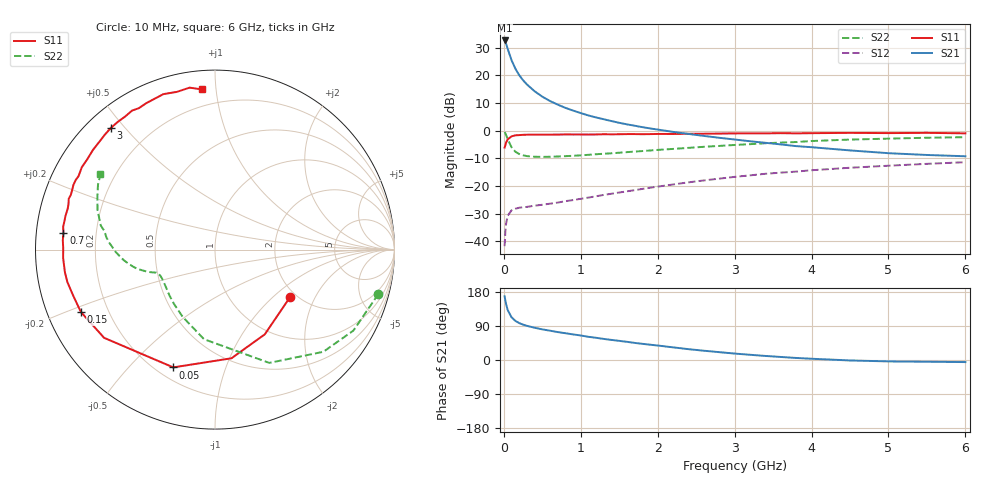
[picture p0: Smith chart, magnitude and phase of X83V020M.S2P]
! SIEMENS Small Signal Semiconductors
! BFP136W
! Si NPN RF Bipolar Junction Transistor in SOT343
! VCE = 3 V  IC = 20 mA
! Common Emitter S-Parameters:  September  1994
# GHz  S  MA  R  50
!  f  S11  S21  S12  S22
! GHz  MAG  ANG  MAG  ANG  MAG  ANG  MAG  ANG
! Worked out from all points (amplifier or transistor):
!   40 points, 10 MHz to 6 GHz, reference 50 ohm
!   highest |S21| = 32.6 dB at 10 MHz (marker M1)
!   |S21| within 3 dB of that: start of sweep to 49.74 MHz
!   unconditionally stable (mu >= 1): 878 MHz to 2.75 GHz
!   at 200 MHz: K = 0.33, MSG = 23.9 dB, |S12| = -27.8 dB
!   at 1.5 GHz: K = 1.15, MAG = 10.2 dB, |S12| = -22.3 dB
!   at 6 GHz: K = 0.99, MSG = 1.1 dB, |S12| = -11.4 dB
!   S11 on the Smith chart (normalised r, x): 10 MHz: 1.84, -1.30; 50 MHz: 0.26, -0.67; 150 MHz: 0.10, -0.22; 700 MHz: 0.08, +0.06; 3 GHz: 0.07, +0.46; 6 GHz: 0.10, +0.92
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0.01  0.4949 -32.6  42.62 168.0  0.0082 76.7  0.9433 -15.2
0.02  0.5477 -59.6  39.7 156.6  0.0153 68.5  0.8935 -30.3
0.03  0.6124 -81.4  36.97 147.0  0.0212 59.6  0.8298 -43.3
0.05  0.6962 -109.5  30.09 132.0  0.029 45.7  0.7 -64.4
0.1  0.7896 -141.5  18.77 112.7  0.0365 31.0  0.5029 -97.0
0.15  0.8242 -155.1  13.2 103.2  0.0389 26.3  0.4167 -115.4
0.2  0.8313 -162.4  10.05 97.4  0.0406 24.5  0.3788 -127.2
0.25  0.8421 -167.6  8.145 93.3  0.0414 24.2  0.3595 -135.1
0.3  0.8456 -171.3  6.83 90.2  0.042 24.8  0.3472 -140.7
0.4  0.8475 -176.8  5.156 85.1  0.0442 26.7  0.3381 -147.8
0.5  0.8457 179.4  4.115 80.8  0.0459 29.4  0.3362 -152.1
0.6  0.8494 176.6  3.432 77.4  0.048 31.7  0.3378 -154.6
0.7  0.8499 173.6  2.958 73.7  0.0502 34.9  0.3415 -156.1
0.9  0.8538 169.5  2.307 67.5  0.0558 39.0  0.3518 -158.6
1.1  0.8518 164.5  1.882 61.2  0.0619 43.0  0.3664 -159.7
1.6  0.8672 155.5  1.302 48.0  0.0802 49.5  0.4095 -163.1
2.2  0.8716 144.7  0.951 33.4  0.1067 51.6  0.4682 -168.5
3  0.8925 130.5  0.693 17.0  0.1464 48.5  0.5518 -178.4
3.2  0.8942 127.2  0.644 13.8  0.1559 47.2  0.5708 178.8
4.5  0.9127 108.4  0.44 -1.2  0.214 36.0  0.6907 161.4
5.5  0.9134 98.9  0.364 -4.6  0.2517 27.7  0.7454 151.0
6  0.895 94.6  0.345 -5.5  0.2697 23.1  0.7638 146.7
